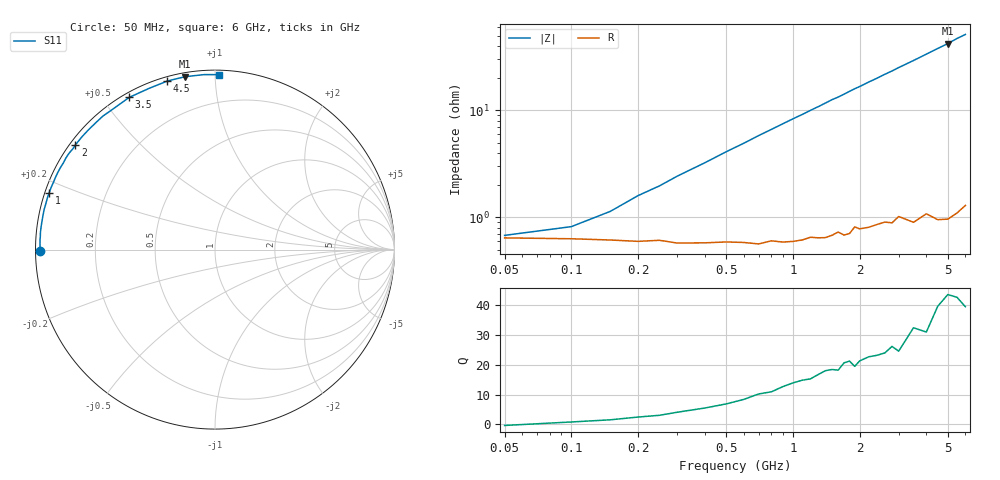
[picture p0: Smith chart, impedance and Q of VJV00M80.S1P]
! Infineon Technologies  Discrete & RF Semiconductors
! BB 914
! Si Tuning Diode in SOT23
! VR =
! S-Parameters:  July  1999
# GHz  S  MA  R  50
!  f  S11
! GHz  MAG  ANG
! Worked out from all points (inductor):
!   34 points, 50 MHz to 6 GHz, reference 50 ohm
!   read as one part to ground: L = 1.25 nH near 250 MHz
!   highest Q = 42.6 at 5 GHz (marker M1), where L = 1.34 nH
!   S11 on the Smith chart (normalised r, x): 50 MHz: 0.01, -0.00; 1 GHz: 0.01, +0.17; 2 GHz: 0.02, +0.33; 3.5 GHz: 0.02, +0.58; 4.5 GHz: 0.02, +0.76; 6 GHz: 0.03, +1.02
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0.05  0.9745 -179.5
0.1  0.975 178.8
0.15  0.9757 177.8
0.2  0.9764 176.6
0.25  0.9758 175.7
0.3  0.9772 174.6
0.5  0.9768 170.7
0.7  0.9779 166.8
0.8  0.9765 164.9
1  0.977 161.1
1.3  0.9756 155.6
1.5  0.9747 151.8
1.6  0.9731 150.2
1.7  0.9749 148.4
1.8  0.9744 146.5
1.9  0.9708 144.7
2  0.9722 143.1
2.2  0.9718 139.6
2.4  0.9707 136.4
2.6  0.97 133.0
2.8  0.9711 130.0
3  0.9679 126.7
3.5  0.9735 119.4
4  0.9706 112.3
4.5  0.976 105.8
5  0.9776 99.9
5.5  0.9768 93.6
6  0.975 88.7
